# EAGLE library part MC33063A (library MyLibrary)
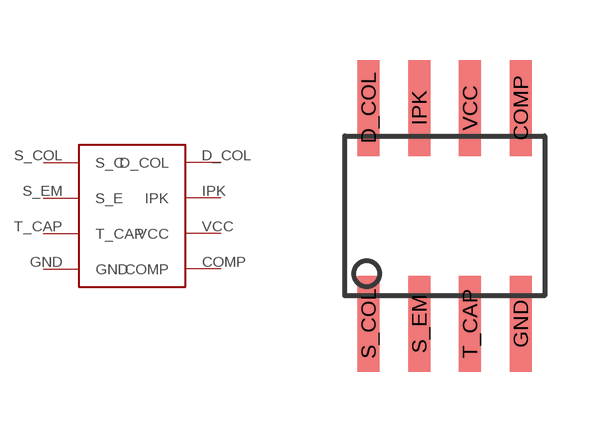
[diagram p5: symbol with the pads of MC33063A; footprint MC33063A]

Designator prefix -

## MC33063A  [MC33063A]
COMP  COMP
D_COL  D_COL
GND  GND
IPK  IPK
S_COL  S_C
S_EM  S_E
T_CAP  T_CAP
VCC  VCC

## Footprint MC33063A (pad centres in mm)
smd 0.55 x 2.4: COMP 1.905,2.7; D_COL -1.905,2.7; GND 1.905,-2.7; IPK -0.635,2.7; S_COL -1.905,-2.7; S_EM -0.635,-2.7; T_CAP 0.635,-2.7; VCC 0.635,2.7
